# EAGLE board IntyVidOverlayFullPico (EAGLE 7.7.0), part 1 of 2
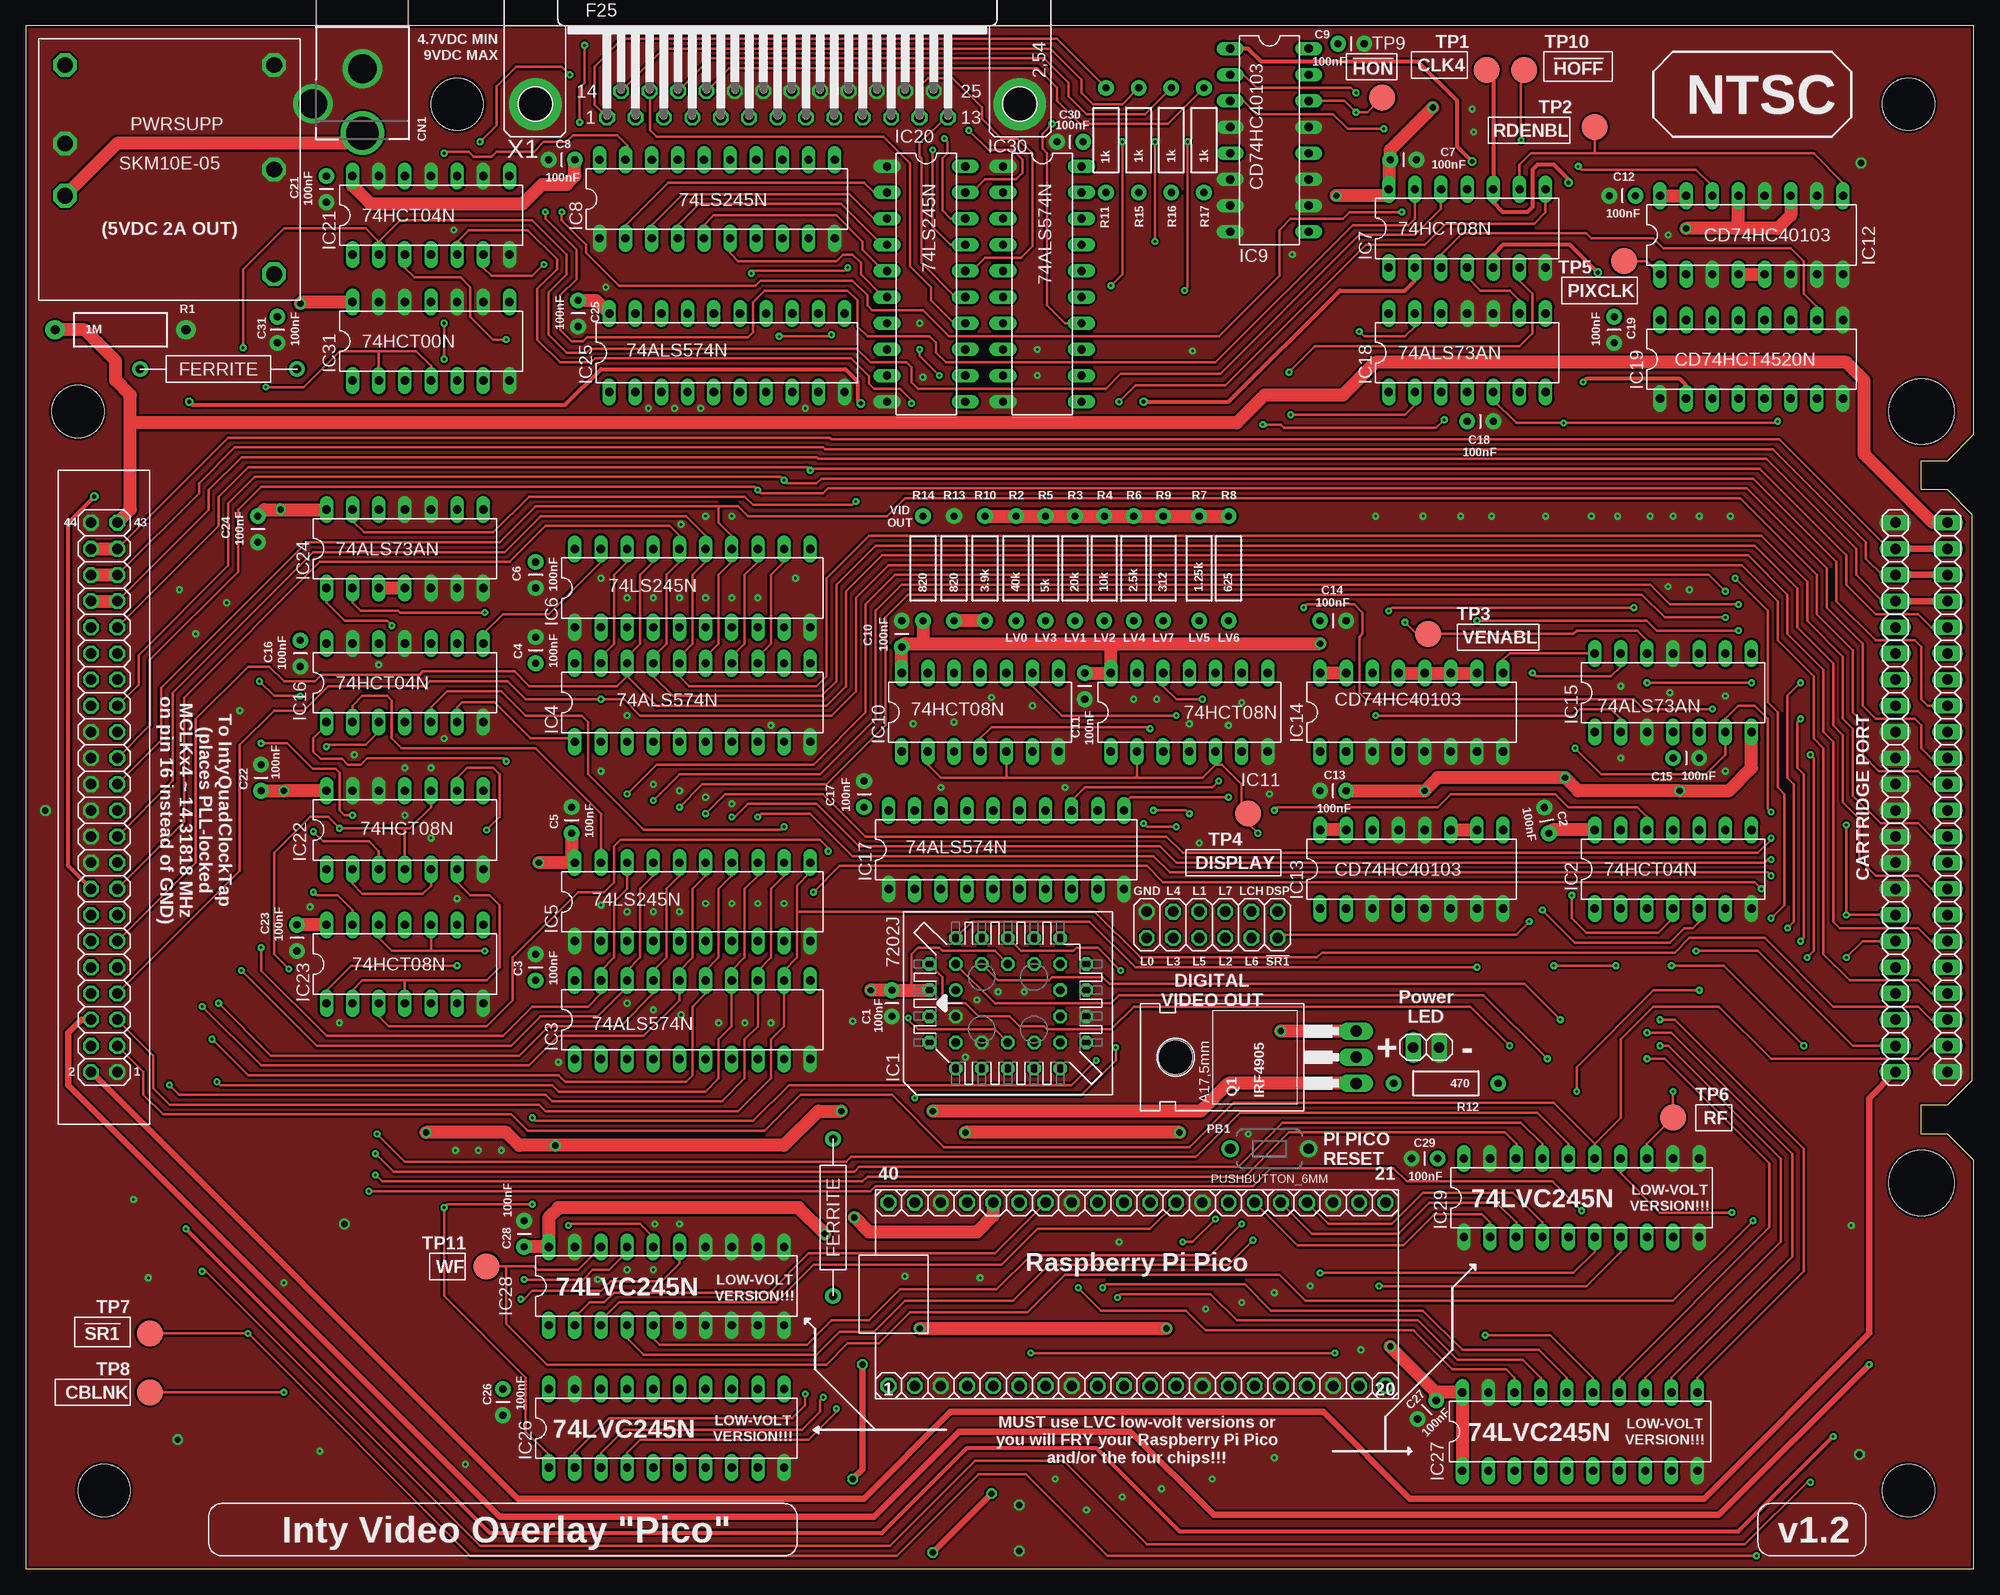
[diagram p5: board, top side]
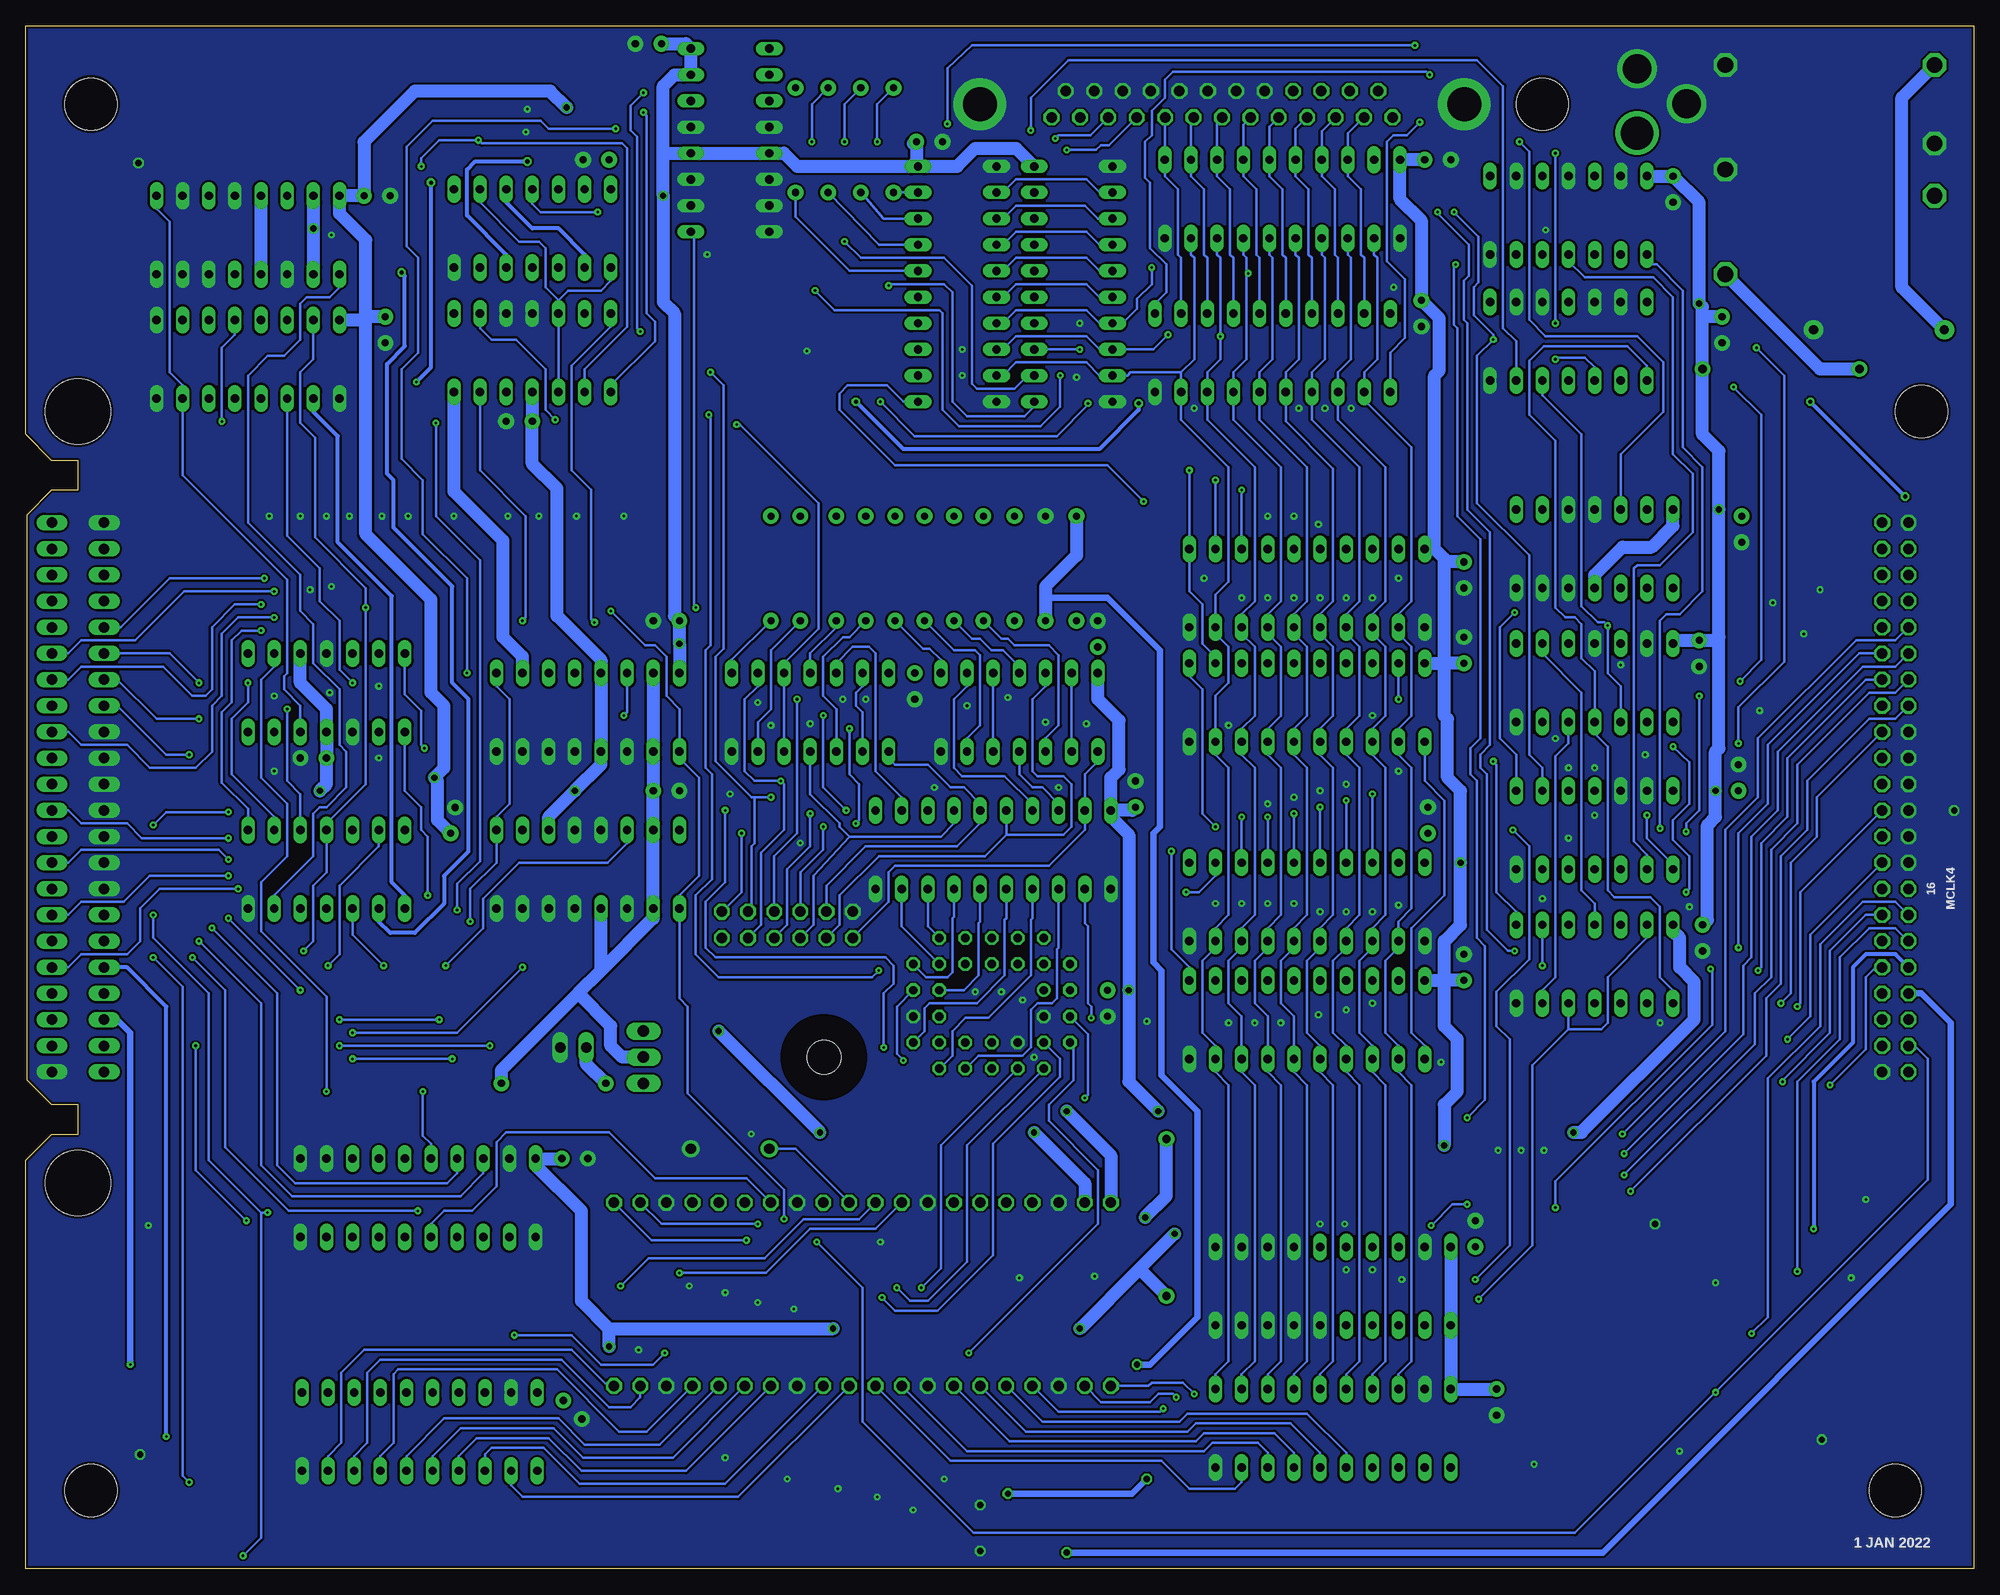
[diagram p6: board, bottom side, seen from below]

Size 189.23 x 149.86 mm. Coordinates in mm from the lower left corner, seen from the top.
Outline: 0,0 189.23,0 189.23,39.69 186.69,42.23 184.15,42.23 184.15,45.09 186.69,45.09 189.07,47.47 189.07,102.39 186.69,104.78 184.15,104.78 184.15,107.63 186.69,107.63 189.23,110.17 189.23,149.86 0,149.86 0,0
Copper layers (1*16): Top 0.035mm / dielectric 1.5mm / Bottom 0.035mm
Design rules "default *": minimum track width 10mil, minimum drill 10mil, track to track 8mil, track to pad 8mil, pad to pad 8mil, via to via 8mil, smd to smd 8mil, copper to edge 10mil, drill to drill 8mil, minimum pad ring 10mil, minimum via ring 8mil, stop-mask expansion 4mil, vias tented up to drill 0mil, thermal gap 10mil
Holes 6.35 mm at 184.15,37.47 184.15,112.39
Holes 5.08 mm at 182.88,7.62 182.88,142.24 7.62,7.62 5.08,112.39 41.91,142.24

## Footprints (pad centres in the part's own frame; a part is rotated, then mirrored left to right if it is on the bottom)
CAP-PTH-SMALL = drill 0.7 pad 1.524: 1 0,0; 2 2.54,0
DCJACK_2MM_PTH = drill 2.8: GND 0,7.35; GNDBREAK 4.8,10.75 | drill 3.2: PWR 0,13.6
FERRITE_0_6 = drill 0.813 pad 1.524: P$1 -7.62,0; P$2 7.62,0
PLCC-S32--SOCKET = drill 0.813: 1 1.27,5.08 | drill 0.813 octagon: 2 -1.27,7.62; 3 -1.27,5.08; 4 -3.81,7.62; 5 -6.35,5.08; 6 -3.81,5.08; 7 -6.35,2.54; 8 -3.81,2.54; 9 -6.35,0; 10 -3.81,0; 11 -6.35,-2.54; 12 -3.81,-2.54; 13 -6.35,-5.08; 14 -3.81,-7.62; 15 -3.81,-5.08; 16 -1.27,-7.62; 17 -1.27,-5.08; 18 1.27,-7.62; 19 1.27,-5.08; 20 3.81,-7.62; 21 6.35,-5.08; 22 3.81,-5.08; 23 6.35,-2.54; 24 3.81,-2.54; 25 6.35,0; 26 3.81,0; 27 6.35,2.54; 28 3.81,2.54; 29 6.35,5.08; 30 3.81,7.62; 31 3.81,5.08; 32 1.27,7.62
DIL14 = drill 0.813 long: 1 -7.62,-3.81; 2 -5.08,-3.81; 3 -2.54,-3.81; 4 0,-3.81; 5 2.54,-3.81; 6 5.08,-3.81; 7 7.62,-3.81; 8 7.62,3.81; 9 5.08,3.81; 10 2.54,3.81; 11 0,3.81; 12 -2.54,3.81; 13 -5.08,3.81; 14 -7.62,3.81
DIL20 = drill 0.813 long: 1 -11.43,-3.81; 2 -8.89,-3.81; 3 -6.35,-3.81; 4 -3.81,-3.81; 5 -1.27,-3.81; 6 1.27,-3.81; 7 3.81,-3.81; 8 6.35,-3.81; 9 8.89,-3.81; 10 11.43,-3.81; 11 11.43,3.81; 12 8.89,3.81; 13 6.35,3.81; 14 3.81,3.81; 15 1.27,3.81; 16 -1.27,3.81; 17 -3.81,3.81; 18 -6.35,3.81; 19 -8.89,3.81; 20 -11.43,3.81
DIL16 = drill 0.813 long: 1 -8.89,-3.81; 2 -6.35,-3.81; 3 -3.81,-3.81; 4 -1.27,-3.81; 5 1.27,-3.81; 6 3.81,-3.81; 7 6.35,-3.81; 8 8.89,-3.81; 9 8.89,3.81; 10 6.35,3.81; 11 3.81,3.81; 12 1.27,3.81; 13 -1.27,3.81; 14 -3.81,3.81; 15 -6.35,3.81; 16 -8.89,3.81
1X20/OCTAGONAL = drill 1.016 octagon: 1 -24.13,0; 2 -21.59,0; 3 -19.05,0; 4 -16.51,0; 5 -13.97,0; 6 -11.43,0; 7 -8.89,0; 8 -6.35,0; 9 -3.81,0; 10 -1.27,0; 11 1.27,0; 12 3.81,0; 13 6.35,0; 14 8.89,0; 15 11.43,0; 16 13.97,0; 17 16.51,0; 18 19.05,0; 19 21.59,0; 20 24.13,0
2X06 = drill 1.016 octagon: 1 -6.35,-1.27; 2 -6.35,1.27; 3 -3.81,-1.27; 4 -3.81,1.27; 5 -1.27,-1.27; 6 -1.27,1.27; 7 1.27,-1.27; 8 1.27,1.27; 9 3.81,-1.27; 10 3.81,1.27; 11 6.35,-1.27; 12 6.35,1.27
2X22 = drill 1.016 octagon: 1 -25.4,-1.27; 2 -25.4,1.27; 3 -22.86,-1.27; 4 -22.86,1.27; 5 -20.32,-1.27; 6 -20.32,1.27; 7 -17.78,-1.27; 8 -17.78,1.27; 9 -15.24,-1.27; 10 -15.24,1.27; 11 -12.7,-1.27; 12 -12.7,1.27; 13 -10.16,-1.27; 14 -10.16,1.27; 15 -7.62,-1.27; 16 -7.62,1.27; 17 -5.08,-1.27; 18 -5.08,1.27; 19 -2.54,-1.27; 20 -2.54,1.27; 21 0,-1.27; 22 0,1.27; 23 2.54,-1.27; 24 2.54,1.27; 25 5.08,-1.27; 26 5.08,1.27; 27 7.62,-1.27; 28 7.62,1.27; 29 10.16,-1.27; 30 10.16,1.27; 31 12.7,-1.27; 32 12.7,1.27; 33 15.24,-1.27; 34 15.24,1.27; 35 17.78,-1.27; 36 17.78,1.27; 37 20.32,-1.27; 38 20.32,1.27; 39 22.86,-1.27; 40 22.86,1.27; 41 25.4,-1.27; 42 25.4,1.27; 43 27.94,-1.27; 44 27.94,1.27
1X22 = drill 1.016 long: 1 -26.67,0; 2 -24.13,0; 3 -21.59,0; 4 -19.05,0; 5 -16.51,0; 6 -13.97,0; 7 -11.43,0; 8 -8.89,0; 9 -6.35,0; 10 -3.81,0; 11 -1.27,0; 12 1.27,0; 13 3.81,0; 14 6.35,0; 15 8.89,0; 16 11.43,0; 17 13.97,0; 18 16.51,0; 19 19.05,0; 20 21.59,0; 21 24.13,0; 22 26.67,0
1X02 = drill 1.016 long: 1 -1.27,0; 2 1.27,0
PUSHBUTTON_6MM = drill 1 pad 1.676: 1 -3.81,0; 2 3.81,0
SKM = drill 1.524 octagon: 1 -10.16,-2.54; 2 -10.16,2.54; 3 10.16,-10.16; 4 10.16,0; 5 10.16,10.16; 6 -10.16,10.16
TO220BH = drill 1.118 long: D 0,-6.35; G -2.54,-6.35; S 2.54,-6.35 | hole 3.302: 0,11.176
AXIAL-0.5 = drill 0.9 pad 1.88: P$1 -6.35,0; P$2 6.35,0
AXIAL-0.4 = drill 0.7 pad 1.524: P$1 -5.08,0; P$2 5.08,0
B2,54 = smd 2.54 x 2.54: TP 0,0
F25HP = drill 1.016 octagon: 1 -16.561,-1.27; 2 -13.792,-1.27; 3 -11.049,-1.27; 4 -8.28,-1.27; 5 -5.512,-1.27; 6 -2.769,-1.27; 7 0,-1.27; 8 2.769,-1.27; 9 5.512,-1.27; 10 8.28,-1.27; 11 11.049,-1.27; 12 13.792,-1.27; 13 16.561,-1.27; 14 -15.189,1.27; 15 -12.421,1.27; 16 -9.652,1.27; 17 -6.909,1.27; 18 -4.14,1.27; 19 -1.372,1.27; 20 1.372,1.27; 21 4.14,1.27; 22 6.909,1.27; 23 9.652,1.27; 24 12.421,1.27; 25 15.189,1.27 | drill 3.302 pad 5.08: G1 -23.52,0; G2 23.52,0

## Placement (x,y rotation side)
C1  100nF  [CAP-PTH-SMALL]  84.14,56.2 270 top
C2  100nF  [CAP-PTH-SMALL]  147.96,71.44 100 top
C3  100nF  [CAP-PTH-SMALL]  49.53,57.15 90 top
C4  100nF  [CAP-PTH-SMALL]  49.53,87.95 90 top
C5  100nF  [CAP-PTH-SMALL]  53.02,71.44 90 top
C6  100nF  [CAP-PTH-SMALL]  49.53,97.79 270 top
C7  100nF  [CAP-PTH-SMALL]  132.56,136.84 0 top
C8  100nF  [CAP-PTH-SMALL]  53.34,136.84 180 top
C9  100nF  [CAP-PTH-SMALL]  127.48,148.11 0 top
C10  100nF  [CAP-PTH-SMALL]  85.09,89.53 90 top
C11  100nF  [CAP-PTH-SMALL]  102.87,87 270 top
C12  100nF  [CAP-PTH-SMALL]  156.37,133.35 180 top
C13  100nF  [CAP-PTH-SMALL]  128.27,75.56 180 top
C14  100nF  [CAP-PTH-SMALL]  125.73,92.08 0 top
C15  100nF  [CAP-PTH-SMALL]  160.02,78.74 0 top
C16  100nF  [CAP-PTH-SMALL]  26.67,90.17 270 top
C17  100nF  [CAP-PTH-SMALL]  81.44,73.98 90 top
C18  100nF  [CAP-PTH-SMALL]  140.02,111.44 0 top
C19  100nF  [CAP-PTH-SMALL]  154.31,121.6 270 top
C21  100nF  [CAP-PTH-SMALL]  29.21,135.25 270 top
C22  100nF  [CAP-PTH-SMALL]  22.86,75.56 90 top
C23  100nF  [CAP-PTH-SMALL]  26.35,62.55 270 top
C24  100nF  [CAP-PTH-SMALL]  22.54,102.23 270 top
C25  100nF  [CAP-PTH-SMALL]  53.66,123.19 270 top
C26  100nF  [CAP-PTH-SMALL]  46.35,17.46 270 top
C27  100nF  [CAP-PTH-SMALL]  137,16.35 225 top
C28  100nF  [CAP-PTH-SMALL]  48.42,31.27 90 top
C29  100nF  [CAP-PTH-SMALL]  137.16,39.85 180 top
C30  100nF  [CAP-PTH-SMALL]  102.71,138.59 180 top
C31  100nF  [CAP-PTH-SMALL]  24.45,121.6 270 top
CN1  [DCJACK_2MM_PTH]  32.7,153.03 180 top
FB1  [FERRITE_0_6]  18.73,116.52 0 top
FB2  [FERRITE_0_6]  78.42,34.13 270 top
IC1  7202J  [PLCC-S32--SOCKET]  95.41,54.93 90 top
IC2  74HCT04N  [DIL14]  160.02,67.94 0 top
IC3  74ALS574N  [DIL20]  64.77,53.34 0 top
IC4  74ALS574N  [DIL20]  64.77,84.14 0 top
IC5  74LS245N  [DIL20]  64.77,64.77 0 top
IC6  74LS245N  [DIL20]  64.77,95.25 0 top
IC7  74HCT08N  [DIL14]  140.02,130.18 0 top
IC8  74LS245N  [DIL20]  67.15,133.03 0 top
IC9  CD74HC40103  [DIL16]  120.81,138.75 270 top
IC10  74HCT08N  [DIL14]  92.71,83.19 0 top
IC11  74HCT08N  [DIL14]  113.03,83.19 0 top
IC12  CD74HC40103  [DIL16]  167.64,129.54 0 top
IC13  CD74HC40103  [DIL16]  134.62,67.94 0 top
IC14  CD74HC40103  [DIL16]  134.62,83.19 0 top
IC15  74ALS73AN  [DIL14]  160.02,85.09 0 top
IC16  74HCT04N  [DIL14]  36.83,86.04 0 top
IC17  74ALS574N  [DIL20]  95.25,69.85 0 top
IC18  74ALS73AN  [DIL14]  140.02,118.11 0 top
IC19  CD74HCT4520N  [DIL16]  167.64,117.47 0 top
IC20  74LS245N  [DIL20]  87.47,124.78 270 top
IC21  74HCT04N  [DIL14]  39.37,131.44 0 top
IC22  74HCT08N  [DIL14]  36.83,71.75 0 top
IC23  74HCT08N  [DIL14]  36.83,58.74 0 top
IC24  74ALS73AN  [DIL14]  36.83,99.06 0 top
IC25  74ALS574N  [DIL20]  68.1,118.11 0 top
IC26  74LVC245N  [DIL20]  62.23,13.65 0 top
IC27  74LVC245N  [DIL20]  150.97,13.34 0 top
IC28  74LVC245N  [DIL20]  62.23,27.46 0 top
IC29  74LVC245N  [DIL20]  151.13,36.04 0 top
IC30  74ALS574N  [DIL20]  98.74,124.78 270 top
IC31  74HCT00N  [DIL14]  39.37,119.22 0 top
JP1  [1X20/OCTAGONAL]  107.95,17.78 0 top
JP2  [1X20/OCTAGONAL]  107.95,35.56 0 top
JP3  [2X06]  115.25,62.55 0 top
JP4  [2X22]  7.62,73.66 90 top
JP5  [1X22]  181.61,74.93 90 top
JP6  [1X22]  186.69,74.93 90 top
JP7  [1X02]  136.05,50.64 0 top
PB1  PUSHBUTTON_6MM  [PUSHBUTTON_6MM]  120.81,40.8 0 top
PWRSUPP  SKM10E-05  [SKM]  13.97,135.89 0 top
Q1  IRF4905  [TO220BH]  122.87,49.69 90 top
R1  1M  [AXIAL-0.5]  9.21,120.33 0 top
R2  40k  [AXIAL-0.4]  96.2,97.16 90 top
R3  20k  [AXIAL-0.4]  101.92,97.16 90 top
R4  10k  [AXIAL-0.4]  104.78,97.16 90 top
R5  5k  [AXIAL-0.4]  99.06,97.16 90 top
R6  2.5k  [AXIAL-0.4]  107.63,97.16 90 top
R7  1.25k  [AXIAL-0.4]  113.98,97.16 90 top
R8  625  [AXIAL-0.4]  116.84,97.16 90 top
R9  312  [AXIAL-0.4]  110.49,97.16 90 top
R10  3.9k  [AXIAL-0.4]  93.19,97.16 270 top
R11  1k  [AXIAL-0.4]  104.93,138.75 90 top
R12  470  [AXIAL-0.4]  137.95,47.15 180 top
R13  820  [AXIAL-0.4]  90.17,97.16 270 top
R14  820  [AXIAL-0.4]  87.15,97.16 270 top
R15  1k  [AXIAL-0.4]  108.11,138.75 270 top
R16  1k  [AXIAL-0.4]  111.28,138.75 270 top
R17  1k  [AXIAL-0.4]  114.46,138.75 270 top
TP1  TPB2,54  [B2,54]  141.92,145.57 0 top
TP2  TPB2,54  [B2,54]  152.4,140.02 0 top
TP3  TPB2,54  [B2,54]  136.21,90.81 0 top
TP4  TPB2,54  [B2,54]  118.75,73.34 0 top
TP5  TPB2,54  [B2,54]  155.26,127 0 top
TP6  TPB2,54  [B2,54]  160.02,43.81 0 top
TP7  TPB2,54  [B2,54]  12.06,22.86 0 top
TP8  TPB2,54  [B2,54]  12.06,17.14 0 top
TP9  TPB2,54  [B2,54]  131.76,142.88 0 top
TP10  TPB2,54  [B2,54]  145.57,145.57 0 top
TP11  TPB2,54  [B2,54]  44.77,29.37 0 top
X1  [F25HP]  73.03,142.24 0 top

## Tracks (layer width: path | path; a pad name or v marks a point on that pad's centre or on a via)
3V3  (via drill 0.61)
  Top 1.27: v110.81,23.34 v86.84,23.34 | IC27.1 IC27.20 137,17.14 | 137,17.14 v132.56,21.59 | C27.1 137,17.14 | v77.63,32.54 75.09,35.08 51.75,35.08 50.8,34.13 IC28.20 C28.1
  Bottom 1.27: 132.56,23.34 135.25,26.04 135.25,34.77 139.7,39.21 IC29.20 C29.1 | 132.56,23.34 v110.81,23.34 | v86.84,23.34 81.04,29.13 | 81.04,29.13 v77.63,32.54 | C26.1 IC26.20 IC28.1 IC28.20 | v132.56,21.59 132.56,23.34 | FB2.P$2 81.04,29.13
3V3SUPP  (via drill 0.61)
  Top 1.27: JP2.5 93.98,34.29 92.39,32.7 81.92,32.7 v80.49,34.13
  Bottom 1.27: v80.49,34.13 78.42,36.2 FB2.P$1
!ACK  (via drill 0.25)
  Top 0.254: IC20.17 89.85,128.59 88.11,130.33 v88.11,137.79
  Bottom 0.254: v88.11,137.79 85.25,137.79 84.77,138.27 84,138.27 X1.10
!AUTOLF  (via drill 0.25)
  Top 0.254: X1.14 61.96,147.64 99.54,147.64 102.55,144.62 102.55,143.35 103.66,142.24 106.52,142.24 R15.P$1 | v109.7,128.91 v109.7,138.59
  Bottom 0.254: IC20.12 91.92,115.89 93.19,114.62 96.84,114.62 97.31,115.09 97.31,124.62 100.01,127.32 108.11,127.32 v109.7,128.91 | v109.7,138.59 109.7,142.24 R15.P$1
!AUTOLF'
  Bottom 0.254: IC30.18 105.89,131.13 R15.P$2
!CBLNK  (via drill 0.25)
  Top 0.254: v163.83,83.5 157.16,83.5 156.21,84.45 130.18,84.45 129.54,85.09 129.54,90.49 129.86,90.81 129.86,92.87 129.06,93.66 124.46,93.66 v124.14,93.34
  Bottom 0.254: IC2.10 162.56,75.25 163.83,76.52 v163.83,83.5 | v124.14,93.34 124.3,93.5 124.3,129.54 IC9.9
!CLK4  (via drill 0.41)
  Top 0.406: v140.49,136.68 139.06,138.11 139.06,142.56 135.25,146.37 120.02,146.37 118.75,147.64 IC9.1 | v152.72,125.89 150.02,128.59 143.51,128.59 142.56,127.64 IC7.5
  Bottom 0.406: IC7.5 142.56,127.64 146.37,131.44 146.37,135.89 145.57,136.68 v140.49,136.68 | v152.72,125.89 152.4,125.57 152.4,118.75 154.15,117 154.15,106.36 153.51,105.73 153.51,101.12 147.8,95.41 147.8,86.04 146.21,84.45 146.21,69.69 148.59,67.31 148.59,64.61 151.45,61.75 153.83,61.75 154.94,62.87 IC2.2
!DISPOFF  (via drill 0.25)
  Top 0.254: v166.37,91.12 158.43,91.12 157.48,92.08 v140.97,92.08
  Bottom 0.254: IC2.8 167.64,73.82 170.18,76.36 170.18,83.19 169.23,84.14 169.23,90.17 168.28,91.12 v166.37,91.12 | v140.97,92.08 140.65,92.39 140.65,102.23 145.1,106.68 IC18.6
!ERROR
  Top 0.254: IC20.14 90.17,120.97 87.95,123.19 87.95,124.46 85.88,126.52 85.88,136.53 83.34,139.06 61.28,139.06 60.64,139.7 60.64,143.47 X1.15
!HOFF  (via drill 0.25)
  Top 0.254: v150.81,136.21 151.13,135.89 162.24,135.89 163.83,134.3 IC12.14 | IC18.2 134.94,113.03 133.99,112.08 v122.87,112.08 | TP10.TP 145.26,145.26 v145.26,138.75 | v106.36,58.1 104.14,60.33 102.08,60.33 101.76,60.01 96.68,60.01 IC1.25
  Bottom 0.254: IC18.2 134.94,116.52 130.81,120.65 130.81,137.95 131.29,138.43 144.94,138.43 v145.26,138.75 149.07,138.75 150.81,137 v150.81,136.21 | v122.87,112.08 122.71,111.92 122.71,89.69 123.19,89.22 123.19,77.79 122.56,77.15 122.56,66.99 124.14,65.41 124.14,59.69 121.92,57.47 107,57.47 v106.36,58.1
!HON  (via drill 0.25)
  Top 0.254: IC9.14 128.11,142.56 v129.22,141.45 130.33,141.45 TP9.TP
  Bottom 0.254: IC18.1 132.4,114.94 128.11,119.22 128.11,121.13 128.91,121.92 128.91,141.13 v129.22,141.45
!INIT  (via drill 0.25)
  Top 0.254: X1.16 66.55,146.69 98.9,146.69 101.28,144.3 101.28,143.03 103.03,141.29 108.74,141.29 R16.P$1 | v86.84,118.43 86.84,117.79 v88.74,115.89 | v112.55,124.14 112.87,124.46 v112.87,138.59
  Bottom 0.254: IC20.13 v86.84,118.43 | v88.74,115.89 88.74,112.87 90.65,110.97 98.58,110.97 100.17,112.55 100.17,121.92 100.49,122.24 110.65,122.24 v112.55,124.14 | v112.87,138.59 112.87,142.24 R16.P$1
!INIT'
  Bottom 0.254: IC30.17 106.36,128.59 R16.P$2
!MSYNC
  Top 0.254: JP4.3 11.43,48.26 11.43,46.04 13.34,44.13 47.15,44.13 48.74,42.55 71.75,42.55 75.25,46.04 84.14,46.04 89.22,40.96 113.03,40.96 117.32,45.24 148.43,45.24 152.4,41.27 | JP6.2 185.1,50.8 183.83,49.53 169.54,49.53 164.47,54.61 158.12,54.61 154.94,51.44 154.94,43.81 152.4,41.27 | 152.4,41.27 IC29.15
!MSYNC'
  Bottom 0.254: JP2.14 119.22,37.94 128.11,37.94 132.56,42.39 142.56,42.39 143.51,41.43 143.51,37.15 145.89,34.77 148.59,34.77 149.86,33.5 IC29.5
!PIXCLK  (via drill 0.25)
  Top 0.254: IC18.5 142.56,113.51 144.78,111.28 v149.38,111.28 170.02,111.28 v170.18,111.44 | IC2.5 162.56,62.87 161.93,62.23 161.13,62.23 159.7,60.8 150.5,60.8 v147.32,63.98
  Bottom 0.254: v170.18,111.44 170.18,118.59 168.91,119.86 IC19.12 | v147.32,63.98 147.32,66.52 145.1,68.74 145.1,97.95 149.38,102.23 v149.38,111.28
!R  (via drill 0.25)
  Top 0.254: IC21.6 44.45,126.36 45.24,125.57 49.21,125.57 v50.32,126.68 | v49.21,43.81 49.53,43.5 70.64,43.5 74.14,46.99 101.6,46.99 v103.98,49.37
  Bottom 0.254: v50.32,126.68 50.48,126.52 50.48,120.81 50.16,120.49 50.16,102.23 47.94,100.01 47.94,80.64 48.9,79.69 48.9,77.15 48.26,76.52 48.26,61.28 47.47,60.48 47.47,45.56 v49.21,43.81 | IC1.18 104.62,54.61 104.62,50.01 v103.98,49.37
!RB0
  Top 0.254: IC5.19 55.88,73.34 49.53,79.69 36.51,79.69 35.56,80.64 35.56,84.3 35.08,84.77 32.7,84.77 31.75,83.82 IC16.2
!RB1
  Top 0.254: IC16.8 44.45,90.81 46.35,92.71 50.8,92.71 55.88,97.79 IC6.19
!RDENBL  (via drill 0.25)
  Top 0.254: IC18.13 134.94,120.65 133.99,119.7 130.02,119.7 v129.54,120.17 | v129.22,143.35 128.75,143.83 119.54,143.83 118.27,145.1 IC9.2
  Bottom 0.254: v129.54,120.17 129.86,120.49 129.86,139.06 130.49,139.7 130.49,142.08 v129.22,143.35
!RESET  (via drill 0.25)
  Top 0.254: v17.14,28.89 17.46,28.89 44.13,2.22 83.98,2.22 92.23,10.48 100.81,10.48 108.9,2.38 167,2.38 173.04,8.41 v173.35,8.41 | v176.85,59.37 178.44,60.96 JP5.6
  Bottom 0.254: v173.35,8.41 173.99,9.05 173.99,56.52 v176.85,59.37 | JP4.12 7.62,62.23 10.16,62.23 13.02,59.37 13.02,51.44 17.14,47.31 v17.14,28.89
!SELA
  Top 0.254: IC22.5 39.37,66.36 38.58,65.56 32.7,65.56 31.75,66.52 IC22.2
  Bottom 0.254: IC21.4 39.37,127 37.78,125.41 31.11,125.41 29.21,123.51 29.21,108.27 27.3,106.36 27.3,100.65 30.48,97.47 32.7,97.47 33.02,97.16 33.02,70.64 31.75,69.37 IC22.2
!SELB  (via drill 0.25)
  Top 0.254: IC23.1 29.21,56.2 31.59,58.58 v41.91,58.58
  Bottom 0.254: v41.91,58.58 IC23.9 | IC23.1 29.21,56.2 30.48,57.47 30.48,64.29 31.43,65.25 34.92,65.25 35.56,65.88 35.56,79.85 36.83,81.12 IC16.4 36.83,87.15 38.1,88.42 38.1,91.76 38.73,92.39 39.69,92.39 40.64,93.34 40.64,109.54 43.18,112.08 43.18,117.32 41.75,118.75 33.66,118.75 31.75,116.84 IC31.1
!SELPRT
  Top 0.254: X1.17 68.34,145.73 98.27,145.73 100.17,143.83 100.17,142.56 102.39,140.34 110.97,140.34 R17.P$1
!SELPRT'
  Bottom 0.254: IC30.16 109.22,126.05 114.46,131.29 R17.P$2
!SR1  (via drill 0.25)
  Top 0.254: IC14.9 143.51,88.27 144.15,88.9 IC15.14 | v150.5,79.69 153.03,77.15 163.19,77.15 165.1,79.06 IC15.6 165.1,82.55 166.37,83.82 167.96,83.82 169.23,82.55 169.23,73.82 v169.54,73.5 | JP5.7 v176.85,63.5 v176.85,72.23 | v168.12,1.27 105.09,1.27 97.16,9.21 92.55,9.21 84.61,1.27 43.18,1.27 v21.59,22.86 TP7.TP | JP3.11 121.92,61.59 144.78,61.59 v146.05,62.87 | v165.74,34.61 158.75,34.61 154.94,38.42 IC29.14
  Bottom 0.254: IC14.9 143.51,85.72 142.24,84.45 142.24,74.3 143.51,73.03 IC13.9 143.51,68.58 146.05,66.04 v146.05,62.87 | v150.5,79.69 150.81,80.01 150.81,83.34 152.4,84.93 IC15.14 | v176.85,72.23 175.58,73.5 v169.54,73.5 | 166.37,34.61 171.45,39.69 171.45,55.88 176.85,61.28 v176.85,63.5 | v168.12,1.27 166.37,3.02 166.37,34.61 | v21.59,22.86 20,24.45 20,47.62 14.92,52.7 14.92,60.64 10.79,64.77 7.62,64.77 JP4.14 | 166.37,34.61 v165.74,34.61
!SR1'  (via drill 0.25)
  Top 0.254: v125.73,28.73 150.34,28.73 152.4,30.8 IC29.6
  Bottom 0.254: v125.73,28.73 117.32,28.73 113.03,33.02 106.68,33.02 JP2.9
!STROBE  (via drill 0.25)
  Top 0.254: X1.1 55.24,142.19 55.24,145.89 57.94,148.59 100.17,148.59 R11.P$2 | v105.41,124.62 106.52,125.73 v106.52,138.59
  Bottom 0.254: IC20.11 91.28,112.87 92.23,111.92 97.79,111.92 99.22,113.35 99.22,123.98 100.01,124.78 105.25,124.78 v105.41,124.62 | v106.52,138.59 106.52,142.24 R11.P$2
!STROBE'
  Bottom 0.254: IC30.19 R11.P$1
!VENABL  (via drill 0.25)
  Top 0.254: IC15.13 154.94,87.63 153.99,86.68 146.69,86.68 v146.37,87 | v131.92,139.86 128.43,139.86 127,141.29 119.54,141.29 118.27,142.56 IC9.3
  Bottom 0.254: v146.37,87 146.37,96.2 150.65,100.49 150.65,105.73 152.72,107.79 152.72,116.52 151.13,118.11 151.13,127.32 152.24,128.43 152.24,138.11 149.7,140.65 139.22,140.65 138.43,139.86 v131.92,139.86
!VOFF  (via drill 0.25)
  Top 0.254: v131.13,82.87 150.34,82.87 150.97,83.5 153.99,83.5 154.94,82.55 IC15.2
  Bottom 0.254: IC14.14 130.81,83.19 v131.13,82.87
!VON  (via drill 0.25)
  Top 0.254: v154.46,58.58 v148.43,58.58
  Bottom 0.254: IC2.3 157.48,61.59 v154.46,58.58 | v148.43,58.58 144.78,62.23 144.78,65.09 141.29,68.58 132.72,68.58 130.81,70.48 IC13.14
!WB  (via drill 0.25)
  Top 0.254: IC21.2 34.29,128.91 | 34.29,128.91 36.35,130.97 49.21,130.97 52.55,127.64 52.55,125.73 50.8,123.98 50.8,119.86 52.55,118.11 54.45,118.11 54.85,118.51 80.72,118.51 82.07,117.16 85.57,117.16 86.04,116.68 86.04,115.25 86.68,114.62 104.93,114.62 106.36,116.05 116.05,116.05 129.54,129.54 134.94,129.54 137.48,132.08 IC7.12 | v31.75,73.18 30.96,73.18 30.48,73.66 30.48,77.31 30.08,77.71 27.86,77.71 25.4,80.17 v22.86,80.17 | v21.11,118.59 21.11,126.21 25.08,130.18 33.02,130.18 34.29,128.91
  Bottom 0.254: IC22.1 29.21,68.42 31.75,70.96 v31.75,73.18 | v22.86,80.17 22.86,83.66 18.41,88.11 18.41,115.89 v21.11,118.59
!WB1
  Top 0.254: IC4.1 53.02,80.64 49.05,80.64 45.56,84.14 42.39,84.14 41.91,83.66 IC16.6
  Bottom 0.254: IC3.1 53.34,50.8 54.61,52.07 54.61,62.23 51.44,65.41 51.44,74.61 53.34,76.52 IC4.1
!WF  (via drill 0.25)
  Top 0.254: v121.28,73.66 121.6,73.98 137.16,73.98 138.43,75.25 148.59,75.25 149.86,73.98 156.53,73.98 157.48,73.03 IC2.12 | v105.89,50.64 105.89,49.37 102.55,46.04 86.68,46.04 v86.36,45.72
  Bottom 0.254: v121.28,73.66 121.28,66.67 123.19,64.77 123.19,60.33 122.24,59.37 105.73,59.37 104.93,58.58 104.93,56.83 105.89,55.88 v105.89,50.64 | v86.36,45.72 86.04,46.04 86.04,51.91 IC1.2
B0
  Top 0.254: IC20.2 82.39,133.67 81.44,134.62 62.39,134.62 58.26,130.49 IC8.2
  Bottom 0.254: IC8.2 58.26,127.64 57.94,127.32 57.94,117.47 59.21,116.2 IC25.2 59.21,113.51 54.61,108.9 54.61,93.98 55.88,92.71 IC6.2 55.88,90.81 54.61,89.53 54.61,82.87 55.88,81.6 IC4.2 55.88,79.06 54.61,77.79 54.61,64.14 55.88,62.87 IC5.2 55.88,60.33 57.15,59.05 57.15,52.07 55.88,50.8 IC3.2 55.88,48.26 54.61,46.99 54.61,20.16 55.88,18.89 IC26.18 | IC20.2 84.93,133.67 86.2,134.94 93.03,134.94 94.3,133.67 IC30.2
B0'  (via drill 0.25)
  Top 0.254: v75.72,16.99 75.72,15.88 74.45,14.61 56.67,14.61 53.34,11.27 IC26.2
  Bottom 0.254: JP1.1 80.17,17.78 79.85,18.1 76.83,18.1 v75.72,16.99
B1
  Top 0.254: IC8.3 60.8,130.49 63.82,133.51 80.01,133.51 82.39,131.13 IC20.3
  Bottom 0.254: IC8.3 60.8,127.64 60.48,127.32 60.48,117.47 61.75,116.2 IC25.3 61.75,111.6 57.15,107 57.15,93.98 58.42,92.71 IC6.3 58.42,90.81 57.15,89.53 57.15,82.87 58.42,81.6 IC4.3 58.42,79.06 57.15,77.79 57.15,63.5 58.42,62.23 IC5.3 58.42,60.33 59.69,59.05 59.69,52.07 58.42,50.8 IC3.3 58.42,48.26 57.15,46.99 57.15,20.16 58.42,18.89 IC26.17 | IC20.3 85.09,131.13 86.36,132.4 93.03,132.4 94.3,131.13 IC30.3
B1'  (via drill 0.25)
  Top 0.254: v77.47,16.67 77.15,16.35 77.15,15.24 75.41,13.49 58.1,13.49 55.88,11.27 IC26.3
  Bottom 0.254: v77.47,16.67 77.79,16.99 79.22,16.99 80.01,16.19 84.77,16.19 JP1.2
B2
  Top 0.254: IC8.4 63.34,130.49 65.41,132.56 79.22,132.56 83.19,128.59 IC20.4
  Bottom 0.254: IC8.4 63.34,127.64 63.02,127.32 63.02,117.47 64.29,116.2 IC25.4 64.29,111.6 59.69,107 59.69,93.98 60.96,92.71 IC6.4 60.96,90.81 59.69,89.53 59.69,82.87 60.96,81.6 IC4.4 60.96,79.06 59.69,77.79 59.69,63.5 60.96,62.23 IC5.4 60.96,60.33 62.23,59.05 62.23,52.07 60.96,50.8 IC3.4 60.96,48.26 59.69,46.99 59.69,20.16 60.96,18.89 IC26.16 | IC20.4 84.93,128.59 86.2,129.86 93.03,129.86 94.3,128.59 IC30.4
B2'  (via drill 0.25)
  Top 0.254: v78.74,15.56 78.74,15.24 76.04,12.54 59.69,12.54 58.42,11.27 IC26.4
  Bottom 0.254: JP1.4 88.9,15.24 79.06,15.24 v78.74,15.56
B3
  Top 0.254: IC20.5 83.34,126.05 81.28,128.11 81.28,128.91 78.74,131.44 66.83,131.44 65.88,130.49 IC8.5
  Bottom 0.254: IC8.5 65.88,127.64 65.56,127.32 65.56,117.47 66.83,116.2 IC25.5 66.83,111.44 62.23,106.84 62.23,93.98 63.5,92.71 IC6.5 63.5,90.81 62.23,89.53 62.23,82.87 63.5,81.6 IC4.5 63.5,79.06 62.23,77.79 62.23,63.5 63.5,62.23 IC5.5 63.5,60.33 64.77,59.05 64.77,52.07 63.5,50.8 IC3.5 63.5,48.26 62.23,46.99 62.23,20.16 63.5,18.89 IC26.15 | IC20.5 84.93,126.05 86.2,127.32 93.03,127.32 94.3,126.05 IC30.5
B3'
  Bottom 0.254: JP1.5 90.49,14.29 77.15,14.29 76.36,15.08 64.77,15.08 60.96,11.27 IC26.5
B4
  Top 0.254: IC8.6 68.42,127.79 69.22,127 78.74,127 79.38,127.64 80.33,127.64 81.12,126.84 81.12,125.73 83.34,123.51 IC20.6
  Bottom 0.254: IC8.6 68.42,127.64 68.1,127.32 68.1,117.47 69.37,116.2 IC25.6 69.37,111.6 64.77,107 64.77,93.98 66.04,92.71 IC6.6 66.04,90.81 64.77,89.53 64.77,82.87 66.04,81.6 IC4.6 66.04,79.06 64.77,77.79 64.77,63.5 66.04,62.23 IC5.6 66.04,60.33 67.31,59.05 67.31,54.93 66.04,53.66 IC3.6 66.04,48.26 64.77,46.99 64.77,20.16 66.04,18.89 IC26.14 | IC20.6 84.93,123.51 86.2,124.78 93.03,124.78 94.3,123.51 IC30.6
B4'
  Bottom 0.254: JP1.6 92.08,13.34 76.36,13.34 75.56,14.13 66.36,14.13 63.5,11.27 IC26.6
B5  (via drill 0.25)
  Top 0.254: v79.85,126.36 79.53,126.05 70.72,126.05 v70.48,125.81
  Bottom 0.254: IC8.7 70.96,127.64 70.64,127.32 70.64,125.97 v70.48,125.81 70.64,125.65 70.64,117.47 71.91,116.2 IC25.7 71.91,111.6 67.31,107 67.31,93.98 68.58,92.71 IC6.7 68.58,90.81 67.31,89.53 67.31,82.87 68.58,81.6 IC4.7 68.58,79.06 67.31,77.79 67.31,63.5 68.58,62.23 IC5.7 68.58,60.33 69.85,59.05 69.85,54.93 68.58,53.66 IC3.7 68.58,48.26 67.31,46.99 67.31,20.16 68.58,18.89 IC26.13 | IC30.7 94.3,120.97 93.03,122.24 86.2,122.24 84.93,120.97 IC20.7 82.71,120.97 81.28,122.4 81.28,123.35 79.85,124.78 v79.85,126.36
B5'
  Bottom 0.254: JP1.7 93.66,12.38 75.56,12.38 74.77,13.18 67.94,13.18 66.04,11.27 IC26.7
B6  (via drill 0.25)
  Top 0.254: v78.26,119.86 78.11,119.7 v73.18,119.7
  Bottom 0.254: IC8.8 73.5,127.64 73.18,127.32 v73.18,119.7 73.18,117.47 74.45,116.2 IC25.8 74.45,111.6 69.85,107 69.85,93.98 71.12,92.71 IC6.8 71.12,90.81 69.85,89.53 69.85,82.87 71.12,81.6 IC4.8 71.12,79.06 69.85,77.79 69.85,63.5 71.12,62.23 IC5.8 71.12,60.33 72.39,59.05 72.39,54.93 71.12,53.66 IC3.8 71.12,48.26 69.85,46.99 69.85,20.16 71.12,18.89 IC26.12 | IC30.8 94.3,118.43 93.03,119.7 86.2,119.7 84.93,118.43 IC20.8 79.69,118.43 v78.26,119.86
B6'
  Bottom 0.254: JP1.9 97.79,11.43 74.77,11.43 73.98,12.22 69.53,12.22 68.58,11.27 IC26.8
B7
  Bottom 0.254: 76.99,116.2 IC25.9 76.99,111.6 72.39,107 72.39,95.89 73.66,94.61 IC6.9 73.66,90.81 72.39,89.53 72.39,86.04 73.66,84.77 IC4.9 73.66,79.06 72.39,77.79 72.39,63.5 73.66,62.23 IC5.9 73.66,60.33 74.93,59.05 74.93,52.07 73.66,50.8 IC3.9 73.66,48.26 72.39,46.99 72.39,20.16 73.66,18.89 IC26.11 | 76.99,116.2 75.72,117.47 75.72,127.32 76.04,127.64 IC8.9 | 76.99,116.2 81.92,116.2 82.23,115.89 IC20.9 84.93,115.89 86.2,117.16 93.03,117.16 94.3,115.89 IC30.9
B7'
  Bottom 0.254: JP1.10 99.38,10.48 78.9,10.48 76.2,7.78 71.75,7.78 71.12,8.41 IC26.9
BC1'
  Top 0.254: JP2.15 123.51,31.43 133.83,31.43 136.84,34.45 141.45,34.45 142.24,33.66 IC29.2
BC1_IN  (via drill 0.25)
  Top 0.254: v33.97,38.26 34.61,37.62 81.28,37.62 81.76,38.1 118.43,38.1 122.71,42.39 143.67,42.39 144.78,41.27 IC29.18 | v172.4,60.96 172.72,61.28 172.72,77.15 172.09,77.79 172.09,82.23 v172.4,82.55
  Bottom 0.254: JP4.32 7.62,85.09 10.16,85.09 17.14,78.11 17.14,72.39 19.68,69.85 19.68,57.47 21.27,55.88 21.27,50.96 v33.97,38.26 | v172.4,60.96 166.37,54.93 166.37,39.21 163.35,36.2 147,36.2 144.78,38.42 IC29.18 | v172.4,82.55 176.53,82.55 180.34,86.36 JP5.16
BC1OUT
  Top 0.254: JP4.41 19.68,109.86 78.11,109.86 78.26,109.7 170.34,109.7 180.97,99.06 JP5.21
  Top 0.61: JP6.21 JP5.21
  Top 1.27: JP4.42 JP4.41
BC2'
  Top 0.254: JP2.16 124.94,32.54 133.35,32.54 136.37,35.56 142.88,35.56 144.78,33.66 IC29.3
BC2_IN  (via drill 0.25)
  Top 0.254: v33.97,40.32 35.72,38.58 80.49,38.58 80.96,39.05 117.79,39.05 122.08,43.34 145.26,43.34 147.32,41.27 IC29.17 | v172.4,86.04 171.13,84.77 171.13,76.83 171.77,76.2 171.77,62.87 v171.13,62.23
  Bottom 0.254: JP4.34 7.62,87.63 10.79,87.63 19.05,79.38 19.05,73.66 21.59,71.12 21.59,59.37 22.38,58.58 22.38,51.91 v33.97,40.32 | v171.13,62.23 164.78,55.88 164.78,39.21 163.04,37.47 148.27,37.47 147.32,38.42 IC29.17 | v172.4,86.04 175.26,88.9 JP5.17
BC2OUT
  Top 0.254: JP4.39 16.83,104.46 16.83,105.41 20.32,108.9 77.47,108.9 77.63,108.74 169.7,108.74 178.75,99.69 178.75,98.11 180.34,96.52 JP5.20
  Top 0.61: JP6.20 JP5.20
  Top 1.27: JP4.40 JP4.39
BDIR'
  Top 0.254: JP2.17 126.52,33.5 132.72,33.5 135.73,36.51 144.46,36.51 147.32,33.66 IC29.4
BDIR_IN  (via drill 0.25)
  Top 0.254: v34.13,42.23 36.83,39.53 79.69,39.53 80.17,40.01 113.67,40.01 117.95,44.29 146.84,44.29 149.86,41.27 IC29.16 | v166.05,96.2 169.23,93.03 169.23,84.14 170.18,83.19 170.18,75.88 170.81,75.25 170.81,64.45 v169.54,63.18 | v162.56,56.2 158.12,56.2 150.65,48.74 v150.65,46.35
  Bottom 0.254: JP4.36 7.62,90.17 11.43,90.17 20.95,80.64 20.95,74.93 24.13,71.75 24.13,52.23 v34.13,42.23 | JP5.18 180.02,91.44 175.26,96.2 v166.05,96.2 | v169.54,63.18 v162.56,56.2 | v150.65,46.35 150.65,42.07 149.86,41.27 IC29.16
BDIROUT
  Top 0.254: JP4.37 17.78,102.87 17.78,104.78 20.95,107.95 76.83,107.95 76.99,107.79 169.07,107.79 177.8,99.06 177.8,96.52 180.34,93.98 JP5.19
  Top 0.61: JP6.19 JP5.19
  Top 1.27: JP4.38 JP4.37
BIDIR  (via drill 0.25)
  Top 0.254: v53.82,140.49 53.82,143.83 54.29,144.3 v54.29,147.96 | IC30.14 100.97,120.97 99.22,122.71 99.22,137.48 98.74,137.95 98.74,139.38 v99.69,140.34
  Bottom 0.254: IC25.1 56.67,118.11 55.24,119.54 55.24,125.25 56.99,127 56.99,138.59 56.36,139.22 55.09,139.22 v53.82,140.49 | v54.29,147.96 97.31,147.96 99.69,145.73 v99.69,140.34
BUSAK  (via drill 0.25)
  Top 0.254: v33.34,36.67 82.07,36.67 82.55,37.15 119.22,37.15 120.97,38.89 132.87,38.89 134.14,37.62 148.27,37.62 v151.13,34.77 | v173.04,59.37 173.67,60.01 173.67,78.74 v173.35,79.06
  Bottom 0.254: JP4.30 7.62,82.55 10.16,82.55 16.19,76.52 16.19,71.75 18.73,69.22 18.73,56.83 20.16,55.4 20.16,49.85 v33.34,36.67 | v151.13,34.77 163.67,34.77 169.86,40.96 169.86,56.2 v173.04,59.37 | v173.35,79.06 175.58,79.06 180.34,83.82 JP5.15
BUSY  (via drill 0.25)
  Top 0.254: IC20.18 89.85,131.13 89.06,131.92 89.06,137 89.53,137.48 89.53,138.59 v89.22,138.91
  Bottom 0.254: v89.22,138.91 88.9,139.22 85.82,139.22 X1.11
CBLNK  (via drill 0.25)
  Top 0.254: v112.39,31.75 113.35,31.75 v115.57,33.97 | JP5.2 177.48,50.8 168.28,60.01 v162.24,60.01 | v132.4,93.03 132.72,93.34 v156.21,93.34 | TP8.TP v25.08,17.14
  Bottom 0.254: IC13.1 125.73,65.41 123.83,67.31 123.83,76.83 125.73,78.74 IC14.1 125.73,83.5 127,84.77 127,88.58 128.11,89.69 129.06,89.69 v132.4,93.03 | IC19.15 161.29,117.47 162.56,116.2 162.56,111.28 161.13,109.86 161.13,100.17 156.21,95.25 v156.21,93.34 156.21,76.2 160.02,72.39 IC2.11 160.02,67.63 161.29,66.36 161.29,60.96 v162.24,60.01 | JP4.4 5.71,50.8 4.45,49.53 4.45,37.78 v25.08,17.14 38.73,3.49 97.16,3.49 107.95,14.29 107.95,27.3 v112.39,31.75 | v115.57,33.97 115.57,36.83 124.94,46.2 124.94,54.61 125.73,55.4 125.73,62.87
  Bottom 0.305: 125.73,62.87 IC13.1
CLEVEL
  Top 1.27: R8.P$2 R7.P$2 R9.P$2 R6.P$2 R4.P$2 R3.P$2 R5.P$2 R2.P$2 R10.P$1
CLK4  (via drill 0.25, 0.41)
  Top 0.406: IC19.2 161.29,114.94 160.66,115.57 151.61,115.57 v151.29,115.25 | v149.86,134.62 149.86,134.94 148.43,136.37 146.84,136.37 146.37,135.89 146.37,132.24 145.89,131.76 143.51,131.76 142.56,132.72 IC7.10 142.56,144.94 TP1.TP | JP4.16 4.13,68.26 4.13,101.6 v6.67,104.14 | v15.88,113.35 16.19,113.03 52.39,113.03 55.88,116.52 79.61,116.52 80.8,115.33 80.8,113.51 v81.12,113.19 | IC7.2 134.94,125.09 133.99,124.14 127.64,124.14 116.84,113.35 v108.58,113.35
  Bottom 0.254: 142.56,132.72 IC7.10
  Bottom 0.406: IC2.1 152.4,65.41 153.67,66.67 153.67,94.46 158.91,99.69 158.91,110.01 161.29,112.39 IC19.2 | IC7.2 134.94,127.64 137.48,130.18 140.02,130.18 142.56,132.72 | v151.29,115.25 149.86,116.68 v149.86,134.62 | v6.67,104.14 v15.88,113.35 | v81.12,113.19 81.12,112.55 84.93,108.74 103.98,108.74 v108.58,113.35
DA0  (via drill 0.25)
  Top 0.254: IC5.18 58.42,66.04 57.15,64.77 57.15,59.37 55.88,58.1 IC3.19 55.88,55.88 54.61,54.61 49.21,54.61 46.35,51.75 29.21,51.75 22.86,58.1 v22.86,60.33 | v165.1,94.93 163.51,96.52 84.45,96.52 81.6,93.66 81.6,83.19 76.52,78.11 61.28,78.11 v58.42,75.25
  Bottom 0.254: JP6.17 185.1,88.9 183.83,90.17 178.59,90.17 173.83,94.93 v165.1,94.93 | v58.42,75.25 IC5.18 | JP4.33 11.11,88.9 20,80.01 20,74.3 22.86,71.44 v22.86,60.33
DA1  (via drill 0.25)
  Top 0.254: IC5.17 60.96,67.31 59.69,66.04 59.69,59.37 58.42,58.1 IC3.18 58.42,56.52 55.56,53.66 50.01,53.66 47.15,50.8 28.26,50.8 v20.95,58.1 | v166.37,93.66 159.7,93.66 157.8,95.57 85.09,95.57 82.55,93.03 82.55,82.55 77.15,77.15 63.5,77.15 v60.96,74.61
  Bottom 0.254: JP6.16 185.1,86.36 183.83,87.63 175.9,87.63 173.04,84.77 171.77,84.77 171.13,85.41 171.13,91.44 168.91,93.66 v166.37,93.66 | v60.96,74.61 IC5.17 | JP4.31 10.48,86.36 18.1,78.74 18.1,73.03 20.64,70.48 20.64,58.42 v20.95,58.1
DA2  (via drill 0.25)
  Top 0.254: IC5.16 63.5,67.31 62.23,66.04 62.23,59.37 60.96,58.1 IC3.17 60.96,55.88 57.78,52.7 50.8,52.7 47.94,49.85 23.81,49.85 v18.73,54.93 | v165.1,92.39 159.23,92.39 157,94.61 85.72,94.61 83.5,92.39 83.5,81.92 77.79,76.2 65.72,76.2 v63.5,73.98
  Bottom 0.254: JP6.14 185.1,81.28 183.83,80.01 179.39,80.01 177.16,77.79 172.72,77.79 171.13,79.38 171.13,83.82 170.18,84.77 170.18,90.81 168.59,92.39 v165.1,92.39 | v63.5,73.98 IC5.16 | JP4.27 15.24,74.93 15.24,71.12 17.78,68.58 17.78,55.88 v18.73,54.93
DA3  (via drill 0.25)
  Top 0.254: IC5.15 66.04,67.31 64.77,66.04 64.77,59.37 63.5,58.1 IC3.16 63.5,55.24 60.01,51.75 51.75,51.75 48.9,48.9 22.86,48.9 v17.14,54.61 | v169.54,70.96 169.54,70.8 168.28,69.53 112.39,69.53 110.81,71.12 81.6,71.12 77.47,75.25 67.94,75.25 v66.04,73.34
  Bottom 0.254: JP6.11 185.1,73.66 183.83,72.39 179.39,72.39 177.96,70.96 v169.54,70.96 | v66.04,73.34 IC5.15 | JP4.21 16.83,65.72 16.83,54.93 v17.14,54.61
DA4  (via drill 0.25)
  Top 0.254: IC5.14 68.58,67.31 67.31,66.04 67.31,59.37 66.04,58.1 IC3.15 66.04,55.88 64.77,54.61 64.77,47.94 64.14,47.31 52.39,47.31 51.75,47.94 21.59,47.94 v18.1,51.44 | v169.54,68.9 169.23,68.9 168.91,68.58 111.76,68.58 110.17,70.17 80.96,70.17 76.83,74.3 70.17,74.3 68.9,73.03 v68.58,73.03
  Bottom 0.254: JP6.9 185.1,68.58 183.83,69.85 170.5,69.85 v169.54,68.9 | v68.58,73.03 IC5.14 | JP4.17 15.88,61.59 15.88,53.66 v18.1,51.44
DA5  (via drill 0.25)
  Top 0.254: IC5.13 71.12,67.31 69.85,66.04 69.85,59.37 68.58,58.1 IC3.14 68.58,52.7 67.31,51.44 67.31,47.62 66.04,46.35 51.75,46.35 51.12,46.99 18.89,46.99 v18.57,47.31 | v169.54,67.31 169.23,67.63 111.12,67.63 109.54,69.22 80.33,69.22 76.2,73.34 71.44,73.34 v71.12,73.03
  Bottom 0.254: JP6.7 185.1,63.5 183.83,64.77 179.71,64.77 177.16,67.31 v169.54,67.31 | v71.12,73.03 IC5.13 | JP4.13 10.48,63.5 13.97,60.01 13.97,52.07 18.57,47.47 v18.57,47.31
DA6  (via drill 0.25)
  Top 0.254: IC5.12 73.66,67.31 72.39,66.04 72.39,59.37 71.12,58.1 IC3.13 71.12,52.7 69.85,51.44 69.85,47.62 67.63,45.4 51.12,45.4 50.48,46.04 14.92,46.04 v13.97,46.99 | v168.59,66.04 167.96,66.67 110.49,66.67 108.9,68.26 79.06,68.26 v76.52,65.72
  Bottom 0.254: JP6.5 185.1,58.42 183.83,59.69 179.39,59.69 178.12,60.96 178.12,64.14 176.21,66.04 v168.59,66.04 | JP4.9 9.53,58.42 10.48,57.47 10.48,50.48 v13.97,46.99 | v76.52,65.72 75.25,65.72 73.66,67.31 IC5.12
DA7
  Top 0.254: IC5.11 76.2,67.63 74.93,66.36 74.93,63.82 | 74.93,63.82 74.93,59.37 73.66,58.1 IC3.12 73.66,52.7 72.39,51.44 72.39,47.62 69.22,44.45 50.48,44.45 49.85,45.09 13.97,45.09 12.38,46.67 12.38,49.85 JP4.5 | JP6.3 185.1,53.34 183.83,54.61 175.58,54.61 168.91,61.28 161.61,61.28 160.18,59.85 125.89,59.85 125.41,59.37 108.27,59.37 103.82,63.82 74.93,63.82
DA8  (via drill 0.25)
  Top 0.254: IC4.19 55.88,88.58 57.15,89.85 57.15,96.52 58.42,97.79 IC6.18 | JP6.4 185.1,55.88 183.83,57.15 177.16,57.15 174.62,59.69 174.62,79.69 173.67,80.64 173.67,86.68 170.18,90.17 170.18,93.98 166.69,97.47 83.82,97.47 80.64,94.3 80.64,85.25 78.26,82.87 59.69,82.87 58.1,84.45 v55.88,84.45 48.58,84.45 46.83,86.2 39.21,86.2 38.73,85.72 29.37,85.72 26.99,83.34 24.13,83.34 20.8,80.01 20.8,67.79 JP4.7
  Bottom 0.254: v55.88,84.45 IC4.19
DA9
  Top 0.254: IC6.17 60.96,97.79 59.69,96.52 59.69,89.85 58.42,88.58 IC4.18 58.42,86.68 | JP6.6 185.1,60.96 183.83,62.23 176.21,62.23 175.58,62.87 175.58,80.33 174.62,81.28 174.62,87.31 171.13,90.81 171.13,94.61 167.32,98.42 83.19,98.42 79.69,94.93 79.69,85.72 77.79,83.82 61.28,83.82 58.42,86.68 | JP4.11 16.51,68.58 16.51,82.55 21.59,87.63 23.65,87.63 25.08,86.2 28.1,86.2 28.73,86.84 38.26,86.84 38.58,87.15 47.47,87.15 48.9,85.72 57.47,85.72 58.42,86.68
DA10
  Top 0.254: JP6.8 185.1,66.04 183.83,67.31 179.71,67.31 178.12,68.9 178.12,72.87 176.53,74.45 176.53,80.96 175.58,81.92 175.58,87.95 172.09,91.44 172.09,95.25 167.96,99.38 82.55,99.38 78.74,95.57 78.74,86.2 77.31,84.77 62.87,84.77 60.96,86.68 IC4.17 60.96,88.58 62.23,89.85 62.23,96.52 63.5,97.79 IC6.16 63.5,100.33 62.55,101.28 50.48,101.28 46.99,97.79 28.57,97.79 15.4,84.61 15.4,72.55 JP4.15
DA11
  Top 0.254: JP6.10 185.1,71.12 183.83,72.39 180.18,72.39 177.48,75.09 177.48,81.6 176.53,82.55 176.53,88.58 173.04,92.08 173.04,95.89 168.59,100.33 81.92,100.33 77.79,96.2 77.79,86.68 76.83,85.72 64.45,85.72 63.5,86.68 IC4.16 63.5,88.58 64.77,89.85 64.77,96.52 66.04,97.79 IC6.15 66.04,100.33 64.14,102.23 50.01,102.23 46.51,98.74 27.94,98.74 14.29,85.09 14.29,76.52 JP4.19
DA12
  Top 0.254: IC4.15 66.04,88.58 67.31,89.85 67.31,96.52 68.58,97.79 IC6.14 68.58,100.33 67.31,101.6 67.31,103.19 | JP6.12 185.1,76.2 183.83,77.47 180.02,77.47 178.44,79.06 178.44,82.23 177.48,83.19 177.48,89.22 173.99,92.71 173.99,96.52 166.53,103.98 85.41,103.98 83.66,102.23 70.17,102.23 69.22,103.19 67.31,103.19 | JP4.23 13.18,80.49 13.18,85.57 27.3,99.69 46.04,99.69 49.53,103.19 67.31,103.19
DA13  (via drill 0.25)
  Top 0.254: IC4.14 68.58,88.58 69.85,89.85 69.85,96.52 71.12,97.79 IC6.13 | JP6.13 185.1,78.74 184.15,79.69 184.15,81.92 183.51,82.55 179.71,82.55 178.44,83.82 178.44,89.85 174.94,93.34 174.94,97.16 167.16,104.93 77.95,104.93 77.47,104.46 71.44,104.46 v71.12,104.78 70.8,105.09 22.86,105.09 20.64,102.87 20.64,96.84 12.06,88.27 12.06,81.92 JP4.25
  Bottom 0.254: v71.12,104.78 IC6.13
DA14  (via drill 0.25)
  Top 0.254: IC4.13 71.12,88.58 72.39,89.85 72.39,96.52 73.66,97.79 IC6.12 | JP6.15 184.78,83.82 184.15,84.45 184.15,89.53 183.51,90.17 179.71,90.17 175.9,93.98 175.9,97.79 167.8,105.89 77.31,105.89 76.83,105.41 73.98,105.41 v73.66,105.73 73.34,106.05 22.23,106.05 19.68,103.5 19.68,97.47 10.95,88.74 10.95,85.88 JP4.29
  Bottom 0.254: IC6.12 v73.66,105.73
DA15  (via drill 0.25)
  Top 0.254: JP6.18 185.1,91.44 183.83,92.71 179.71,92.71 176.85,95.57 176.85,98.42 168.43,106.84 76.36,106.84 v76.2,106.68 75.88,107 21.59,107 18.73,104.14 18.73,101.28 JP4.35
  Bottom 0.254: v76.2,106.68 IC6.11 76.2,94.93 74.93,93.66 74.93,89.85 73.66,88.58 IC4.12
DISPLAY  (via drill 0.25)
  Top 0.254: IC10.2 87.63,78.11 88.9,76.83 95.25,76.83 | 95.25,76.83 IC10.5 | 95.25,76.83 107.95,76.83 | 107.95,76.83 114.3,76.83 115.57,78.11 | 115.57,78.11 IC11.5 | IC11.2 107.95,76.83 | IC7.4 140.02,125.41 141.29,124.14 144.15,124.14 145.1,123.19 IC18.9 | v120.17,111.12 121.92,111.12 122.24,110.81 137,110.81 v137.79,111.6 | 115.57,78.11 116.2,78.11 118.11,76.2 118.11,73.66 TP4.TP 118.75,72.39 v119.7,71.44
  Bottom 0.254: IC10.5 IC10.10 | IC11.2 107.95,83.19 108.58,83.82 108.58,85.09 107.95,85.72 IC11.13 | IC11.5 IC11.10 115.57,87.95 112.24,91.28 112.24,103.5 119.86,111.12 v120.17,111.12 | IC10.2 IC10.13 | v119.7,71.44 119.7,65.72 JP3.12 | v137.79,111.6 138.75,112.55 138.75,116.52 141.6,119.38 143.99,119.38 145.1,120.49 IC18.9
DISPOFF  (via drill 0.25)
  Top 0.254: v167.64,86.04 v157.48,86.04
  Bottom 0.254: IC2.9 165.1,73.03 169.23,77.15 169.23,82.55 167.64,84.14 v167.64,86.04 | v157.48,86.04 158.75,87.31 158.75,92.08 160.66,93.98 160.66,97.16 163.83,100.33 IC19.3
EXTAUD  (via drill 0.25)
  Top 0.61: JP4.6 5.4,53.34 4.13,52.07 4.13,46.99 46.04,5.08 82.39,5.08 90.65,13.34 107.31,13.34 115.41,5.24 164.47,5.24 v179.07,19.84
  Bottom 0.61: v179.07,19.84 179.07,52.07 180.34,53.34 JP5.3
EXTVID  (via drill 0.61)
  Top 0.61: v81.28,19.84 81.28,9.68 v80.33,8.73 | v93.82,7.3 v88.11,1.59
  Top 1.27: R10.P$2 R13.P$2
  Bottom 0.61: JP4.8 5.08,55.88 2.22,53.02 2.22,35.4 36.04,1.59 v88.11,1.59 | v80.33,8.73 81.76,7.3 v93.82,7.3 | v81.28,19.84 80.01,19.84 75.41,24.45 75.41,44.45 78.9,47.94 78.9,58.1 79.69,58.9 79.69,71.44 79.06,72.07 79.06,89.22 84.14,94.3 90.01,94.3 90.17,94.14
  Bottom 1.27: R14.P$1 87.15,98.42 90.17,95.41 90.17,94.14 R13.P$2
EXTVID2
  Top 0.61: JP4.2 47.78,6.83 81.44,6.83 89.85,15.24 126.05,15.24 134.46,6.83 163.04,6.83 179.07,22.86 179.07,45.72 JP5.1
F0  (via drill 0.25)
  Top 0.254: v102.23,27.3 104.46,25.08 112.71,25.08 114.62,23.18 134.78,23.18 138.59,19.37 143.83,19.37 144.62,18.57 IC27.18
  Bottom 0.254: v102.23,27.3 100.33,29.21 100.33,41.12 IC1.7
F0'
  Bottom 0.254: JP1.11 120.02,6.99 140.97,6.99 142.08,8.1 IC27.2
F1  (via drill 0.25)
  Top 0.254: v106.05,26.35 106.36,26.67 115.09,26.67 117.63,24.13 135.25,24.13 139.06,20.32 145.41,20.32 147.16,18.57 IC27.17
  Bottom 0.254: v106.05,26.35 104.78,25.08 100.65,25.08 95.25,30.48 95.25,41.27 88.74,47.78 88.74,49.53 IC1.6
F1'
  Bottom 0.254: JP1.12 121.28,8.26 135.41,8.26 138.91,11.75 143.99,11.75 144.62,11.11 IC27.3
F2  (via drill 0.25)
  Top 0.254: v104.62,27.3 104.93,27.62 118.43,27.62 120.97,25.08 135.73,25.08 139.54,21.27 147,21.27 149.7,18.57 IC27.16
  Bottom 0.254: v104.62,27.3 103.35,26.04 101.6,26.04 97.79,29.84 97.79,41.12 IC1.5
F2'
  Bottom 0.254: JP1.14 125.09,9.53 135.25,9.53 138.43,12.7 145.41,12.7 147.16,10.95 IC27.4
F3  (via drill 0.25)
  Top 0.254: v127.16,20.95 v97.63,20.95 | v141.76,22.7 148.11,22.7 152.24,18.57 IC27.15
  Bottom 0.254: v141.76,22.7 136.21,22.7 133.35,19.84 128.27,19.84 v127.16,20.95 | v97.63,20.95 85.09,33.5 85.09,38.73 89.85,43.5 89.85,45.09 87.47,47.47 87.47,50.8 IC1.4
F3'
  Bottom 0.254: JP1.15 126.36,10.79 135.1,10.79 137.95,13.65 147,13.65 149.7,10.95 IC27.5
F4  (via drill 0.25)
  Top 0.254: v157.48,49.53 159.23,49.53 169.39,39.37 169.39,33.18 154.78,18.57 IC27.14 | v147.8,49.53 141.6,55.72 106.2,55.72 105.41,54.93 94.14,54.93 IC1.31
  Bottom 0.254: v157.48,49.53 v147.8,49.53
F4'
  Bottom 0.254: JP1.16 127.64,12.06 134.94,12.06 137.48,14.61 148.59,14.61 152.24,10.95 IC27.6
F5  (via drill 0.25)
  Top 0.254: v158.75,50.8 159.54,50.8 170.5,39.85 170.5,31.75 157.32,18.57 IC27.13 | v144.15,50.8 140.34,54.61 107.63,54.61 105.41,52.39 99.22,52.39 98.9,52.7 96.52,52.7 95.57,53.66 92.55,53.66 91.28,54.93 89.53,54.93 89.06,55.4 89.06,57.47 IC1.30
  Bottom 0.254: v158.75,50.8 v144.15,50.8
F5'
  Bottom 0.254: JP1.17 128.91,13.34 131.6,13.34 137.64,19.37 153.03,19.37 153.51,18.89 153.51,12.22 154.78,10.95 IC27.7
F6  (via drill 0.25)
  Top 0.254: v157.48,52.07 159.86,52.07 171.61,40.32 171.61,30.32 159.86,18.57 IC27.12 | v140.97,58.42 107.79,58.42 103.35,62.87 91.92,62.87 IC1.29
  Bottom 0.254: v157.48,52.07 147.32,52.07 v140.97,58.42
F6'
  Bottom 0.254: JP1.19 129.54,16.67 130.49,15.72 132.56,15.72 137.16,20.32 154.78,20.32 156.05,19.05 156.05,12.22 157.32,10.95 IC27.8
F7  (via drill 0.25)
  Top 0.254: v158.75,53.34 160.18,53.34 172.72,40.8 172.72,28.89 162.4,18.57 IC27.11 | v149.07,53.34 145.57,56.83 105.25,56.83 104.62,57.47 99.69,57.47 99.38,57.15 94.46,57.15 IC1.28
  Bottom 0.254: v158.75,53.34 v149.07,53.34
F7'
  Bottom 0.254: JP1.20 132.72,17.78 136.21,21.27 156.37,21.27 158.59,19.05 158.59,12.22 159.86,10.95 IC27.9
G0  (via drill 0.25)
  Top 0.254: v85.72,53.5 85.72,53.34 86.68,52.39 94.14,52.39 IC1.10
  Bottom 0.254: IC17.2 86.36,62.71 86.04,62.39 86.04,54.93 85.72,54.61 v85.72,53.5
G1
  Bottom 0.254: IC17.3 88.9,60.33 89.06,60.17 89.06,55.4 89.53,54.93 90.96,54.93 91.6,54.29 91.6,50.64 92.39,49.85 96.68,49.85 IC1.11
G2
  Bottom 0.254: IC17.4 91.44,63.18 91.6,63.02 91.6,57.63 95.73,53.5 97.95,53.5 99.22,52.23 99.22,49.85 IC1.13
G3
  Bottom 0.254: IC17.5 93.98,63.18 94.14,63.02 94.14,57.63 96.84,54.93 101.44,54.93 101.92,54.45 101.92,52.23 IC1.14
G4
  Bottom 0.254: IC17.6 96.52,62.87 96.68,62.71 96.68,57.63 98.11,56.2 IC1.19
G5
  Bottom 0.254: IC17.7 99.06,63.34 99.22,63.18 99.22,57.94 99.69,57.47 101.76,57.47 IC1.20
G6
  Bottom 0.254: IC17.8 101.6,62.39 IC1.21
G7
  Bottom 0.254: IC17.9 104.14,62.39 IC1.22
GND  (via drill 0.25, 0.61)
  other vias: 118.11,84.14 97.79,83.82 90.17,82.23 88.9,75.88 55.88,77.47 58.42,82.87 66.04,102.23 178.28,136.53 154.62,102.23 157.8,102.23 154.94,78.74 165.1,77.47 67.31,53.02 69.85,53.02 72.39,53.02 51.75,49.21 31.91,79.06 55.88,96.2 63.66,101.44 159.54,129.54 165.1,84.77 159.7,85.09 154.94,85.72 68.58,102.23 107.63,84.45 55.88,64.45 58.42,63.82 60.96,63.82 63.5,63.82 66.04,64.61 68.58,64.61 71.12,64.61 58.42,94.3 60.96,94.3 63.5,94.3 66.04,94.3 68.58,94.3 71.12,94.3 58.42,54.93 60.96,54.29 60.96,76.2 63.5,75.56 66.04,74.93 68.58,74.3 72.39,81.92 14.76,12.54 178.12,11.11 116.84,81.92 109.86,84.45 100.97,75.88 113.98,70.48 92.39,55.24 94.46,56.04 97,56.04 91.28,49.69 63.5,33.5 61.12,33.5 60.96,29.05 58.42,29.05 55.56,28.1 36.83,77.79 39.37,77.79 40.64,80.64 39.37,70.96 36.83,73.18 41.91,65.09 34.29,87.79 60.48,112.71 63.02,112.71 65.56,112.71 75.72,112.71 56.36,124.46 41.59,130.02 98.27,118.43 98.27,115.89 86.84,120.97 96.52,6.19 131.13,102.23 135.73,102.23 139.38,102.23 142.4,102.23 152.08,102.23 160.02,102.23 162.56,102.23 165.58,102.23 1.91,73.66 120.81,75.25 93.82,84.61 73.66,64.61 63.66,53.82 106.2,31.75 114.62,25.24 118.11,25.88 121.28,26.83 124.78,27.46 129.7,21.27 96.52,1.75 103.03,5.71 106.52,6.99 110.33,7.78 115.25,8.73 121.28,10.79 30.96,33.5 10.48,35.88 11.91,28.26 28.57,11.43 177.32,33.34 74.77,96.2 14.92,95.09 16.51,90.81 19.53,93.82 20.8,83.34 86.2,82.07 113.03,82.07 161.61,95.09 159.54,95.41 80.33,53.18 46.2,40.64 41.75,40.64 43.97,40.64 140.49,141.76 140.65,139.54 30.48,53.02 27.62,64.29 25.08,27.78 42.7,10.16 100.01,8.73 118.75,42.23 85.41,28.42 92.71,28.26 113.35,118.27 147.64,102.23 123.03,127.64 87.15,115.73
  pour Top (no thermals): -5.08,157.48 208.28,157.48 208.28,-5.08 -5.08,-5.08
  pour Bottom (no thermals): -7.62,160.02 210.82,160.02 210.82,-7.62 -7.62,-7.62
L0
  Bottom 0.254: IC10.1 85.09,78.42 86.36,77.15 IC17.19 86.36,71.75 89.85,68.26 104.78,68.26 105.41,67.63 105.41,64.77 JP3.1
L1  (via drill 0.25)
  Top 0.254: v111.76,72.07 108.9,72.07 v108.58,72.39 | v109.22,81.6 109.06,81.76 93.82,81.76 92.71,80.64 IC10.4
  Bottom 0.254: IC17.18 88.9,74.3 90.49,75.88 91.44,75.88 92.71,77.15 IC10.4 | JP3.6 113.98,67.63 111.76,69.85 v111.76,72.07 | v108.58,72.39 108.27,72.71 108.27,76.2 109.22,77.15 v109.22,81.6
L2  (via drill 0.25)
  Top 0.254: v113.03,73.34 112.71,73.66 v109.54,73.66 | v111.76,82.87 100.65,82.87 97.79,85.72 IC10.9
  Bottom 0.254: IC17.17 91.44,74.3 94.14,76.99 98.27,76.99 99.06,77.79 99.06,84.45 97.79,85.72 IC10.9 | JP3.7 115.25,62.55 115.25,67.94 113.03,70.17 v113.03,73.34 | v109.54,73.66 111.76,75.88 v111.76,82.87
L3
  Bottom 0.254: IC17.16 93.98,71.28 | 93.98,71.28 88.42,71.28 87.63,72.07 87.63,76.2 88.42,76.99 90.96,76.99 91.44,77.47 91.44,84.45 90.17,85.72 IC10.12 | 93.98,71.28 96.04,69.22 106.36,69.22 110.17,65.41 110.17,62.55 JP3.3
L4
  Bottom 0.254: IC11.1 105.41,78.74 104.78,78.11 101.6,78.11 99.38,75.88 98.11,75.88 96.52,74.3 IC17.15 96.52,72.39 98.74,70.17 107.63,70.17 111.44,66.36 JP3.4
L5
  Bottom 0.254: IC17.14 99.06,72.39 100.33,71.12 109.22,71.12 | 109.22,71.12 110.17,72.07 110.17,72.39 113.03,75.25 IC11.4 | JP3.5 112.71,62.55 112.71,67.31 109.22,71.12
L6  (via drill 0.25)
  Top 0.254: IC17.13 101.6,74.61 102.87,75.88 115.25,75.88 v115.89,76.52
  Bottom 0.254: IC11.9 118.11,85.72 119.38,84.45 119.38,77.47 118.43,76.52 v115.89,76.52 115.57,76.2 115.57,71.75 117.79,69.53 117.79,62.55 JP3.9
L7  (via drill 0.25)
  Top 0.254: v114.3,84.45 111.76,84.45 110.49,85.72 IC11.12
  Bottom 0.254: IC11.12 110.49,87.95 108.9,89.53 107.31,89.53 106.68,88.9 106.68,77.47 104.14,74.93 IC17.12 | JP3.8 116.52,69.22 114.3,71.44 v114.3,84.45
LATCH  (via drill 0.25)
  Top 0.254: IC7.6 145.1,125.09 146.37,123.83 146.37,120.02 145.1,118.75 125.25,118.75 v122.71,116.2 | v116.84,74.93 107.31,74.93 106.68,74.3 IC17.11
  Bottom 0.254: v122.71,116.2 121.44,114.94 121.44,89.38 122.24,88.58 122.24,78.42 118.75,74.93 118.43,74.93 | 118.43,74.93 v116.84,74.93 | JP3.10 118.75,64.14 118.75,70.17 118.43,70.48 118.43,74.93
LV0
  Bottom 0.254: IC10.3 90.17,80.64 88.9,81.92 88.9,88.74 89.85,89.69 93.19,89.69 93.82,90.33 94.46,90.33 R2.P$1
LV1
  Bottom 0.254: IC10.6 97.79,80.64 96.52,81.92 96.52,88.74 97,89.22 99.06,89.22 R3.P$1
LV2
  Bottom 0.254: IC10.8 100.33,88.27 101.44,89.38 102.08,89.38 R4.P$1
LV3
  Bottom 0.254: IC10.11 92.71,87.63 94.3,89.22 95.41,89.22 96.52,90.33 97.31,90.33 R5.P$1
LV4
  Bottom 0.254: IC11.3 110.49,83.5 111.76,84.77 111.76,88.58 109.86,90.49 109.22,90.49 R6.P$1
LV5
  Bottom 0.254: IC11.6 118.11,82.23 116.84,83.5 116.84,89.22 R7.P$1
LV6
  Bottom 0.254: IC11.8 120.65,88.27 R8.P$1
LV7
  Bottom 0.254: IC11.11 113.03,88.9 110.49,91.44 R9.P$1
MCLK  (via drill 0.25)
  Top 0.406: v15.56,33.02 45.09,3.49 83.19,3.49 91.44,11.75 103.98,11.75 112.08,3.65 166.37,3.65 v175.58,12.86
  Bottom 0.406: v175.58,12.86 175.58,54.61 179.39,58.42 JP5.5 | JP4.10 7.62,59.69 10.48,59.69 11.75,58.42 11.75,51.12 15.56,47.31 v15.56,33.02
PD0
  Bottom 0.254: X1.2 60.8,139.4 IC8.18 60.8,135.25 59.53,133.99 59.53,127.64 59.21,127.32 IC25.19
PD1
  Bottom 0.254: X1.3 63.34,139.6 IC8.17 63.34,135.25 62.07,133.99 62.07,127.64 61.75,127.32 IC25.18
PD2
  Bottom 0.254: X1.4 65.88,139.83 IC8.16 65.88,135.25 64.61,133.99 64.61,127.64 64.29,127.32 IC25.17
PD3
  Bottom 0.254: X1.5 68.42,140.06 IC8.15 68.42,135.25 67.15,133.99 67.15,127.64 66.83,127.32 IC25.16
PD4
  Bottom 0.254: X1.6 70.96,140.26 IC8.14 70.96,135.25 69.69,133.99 69.69,127.64 69.37,127.32 IC25.15
PD5
  Bottom 0.254: X1.7 73.5,140.49 IC8.13 73.5,135.25 72.23,133.99 72.23,127.64 71.91,127.32 IC25.14
PD6
  Bottom 0.254: X1.8 76.04,140.72 IC8.12 76.04,135.25 74.77,133.99 74.77,127.64 74.45,127.32 IC25.13
PD7
  Bottom 0.254: X1.9 78.58,140.93 IC8.11 78.58,135.25 77.31,133.99 77.31,127.64 76.99,127.32 IC25.12
PIXCLK
  Top 0.254: TP5.TP 157.48,127 IC12.1
  Bottom 0.254: IC12.1 158.75,124.46 159.7,123.51 161.93,123.51 162.56,122.87 162.56,119.38 164.15,117.79 165.74,117.79 167.64,115.89 167.64,101.6 162.56,96.52 162.56,93.03 161.29,91.76 161.29,87.95 158.75,85.41 158.75,80.01 158.12,79.38 158.12,75.88 160.02,73.98 160.66,73.98 161.29,73.34 161.29,69.22 165.1,65.41 IC2.6
POUT
  Top 0.254: IC20.16 91.92,126.05 93.19,127.32 96.68,127.32 97.79,128.43 97.79,137.48 96.36,138.91 94.77,138.91 92.87,140.81 92.87,141.92 90.01,144.78 87.63,144.78 86.84,143.99 86.84,140.99 X1.12
PWR
  Top 1.27: CN1.PWR 31.75,138.43 8.89,138.43 PWRSUPP.1
PWRLED
  Bottom 1.27: R12.P$2 134.78,49.05 JP7.1
R  (via drill 0.25)
  Top 0.254: IC21.5 41.91,128.91 43.02,130.02 48.74,130.02 51.59,127.16 51.59,126.21 49.69,124.3 49.69,119.38 51.91,117.16 54.93,117.16 55.32,117.55 80.17,117.55 81.92,115.81 81.92,115.09 82.39,114.62 84.93,114.62 86.04,113.51 v86.04,113.19 | v106.2,113.35 107.79,114.94 116.52,114.94 130.18,128.59 135.89,128.59 137.95,130.65 146.53,130.65 147.64,131.76 IC7.8
  Bottom 0.254: v86.04,113.19 86.04,113.03 89.06,110.01 102.87,110.01 v106.2,113.35
RB0  (via drill 0.25)
  Top 0.254: v46.67,78.42 46.35,78.74 33.18,78.74 32.54,78.11 31.27,78.11 30.72,78.66 28.65,78.66 27.94,79.38 27.94,80.64 29.21,81.92 IC16.1
  Bottom 0.254: IC23.8 44.45,63.82 46.35,65.72 46.35,78.11 v46.67,78.42
RB1
  Bottom 0.254: IC23.11 36.83,64.61 38.1,65.88 38.1,85.09 41.91,88.9 IC16.9
RDBUS  (via drill 0.25)
  Top 0.254: IC23.12 34.29,61.28 35.56,60.01 39.37,60.01 | 39.37,60.01 IC23.10 | 39.37,60.01 v44.61,60.01 | v52.07,131.76 52.07,130.97 54.45,128.59 54.45,127.79 57.63,124.62 70.88,124.62 71.36,125.09 80.33,125.09 81.76,123.67 81.76,122.71 82.23,122.24 87.15,122.24 89.69,119.7 115.89,119.7 121.76,125.57 121.76,130.02 122.87,131.13 127.95,131.13 128.59,131.76 v133.67,131.76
